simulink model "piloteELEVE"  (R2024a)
settings: Solver=ode45  StartTime=0.0  StopTime=10  RelTol=1e-3  EnableMultiTasking=on
PreLoadFcn:
  | M=0
InitFcn:
  | modelename = gcs
  | path = strcat(modelename,'/mecanisme pilote/Mass')
  | if M==0
  |     set_param(path,'Commented','on')
  | else
  |     set_param(path,'Commented','off')
  | end
libraries: fl_lib x15, nesl_utility x4, sdl_lib x1

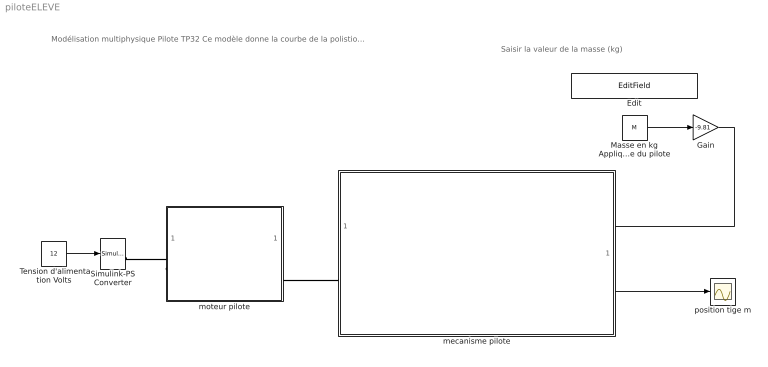
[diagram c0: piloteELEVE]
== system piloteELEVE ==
  note: Saisir la valeur de la masse (kg)
  note: Modélisation multiphysique Pilote TP32 Ce modèle donne la courbe de la polistion de la tige du pilote pendant son mouvement de sortie. Vous pouvez modifier la charge sur la motorisation du pilote en modifiant la valeur de la masse appliquée sur la tige du pilote. Vous devez modifier les paramètres pour que le modèle soit conforme au système.
  " Tension d'alimentation Volts" : Constant  Value=12
  Edit : EditField  LabelPosition=Hide  ShowInitialText=on  Alignment=Center
  Gain : Gain  Gain=-9.81
  Masse en kg Appliquée sur la tige en sortie du pilote : Constant  Value=M
  Simulink-PS Converter : nesl_utility/Simulink-PS Converter  PhysicalDomain=network_engine_domain  SubClassName=ps_input  LeftPortType=input  RightPortType=output  PseudoPeriodic=off  Frequencies=[]  NoiseDistribution=none  NoiseParameters=[]  Unit=1  AffineConversion=off  FilteringAndDerivatives=zero  SimscapeFilterOrder=1  InputFilterTimeConstant=0.001  UdotUserProvided=1
  mecanisme pilote : Subsystem
  moteur pilote : Subsystem
  position tige m : Scope
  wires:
  " Tension d'alimentation Volts"/1 -> Simulink-PS Converter/1
  mecanisme pilote/1(position tige) -> position tige m/1
  Masse en kg Appliquée sur la tige en sortie du pilote/1 -> Gain/1
  Gain/1 -> mecanisme pilote/1(Masse accrochée sur la tige)
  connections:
  moteur pilote/LConn1 -- Simulink-PS Converter/RConn1
  moteur pilote/RConn1 -- mecanisme pilote/LConn1

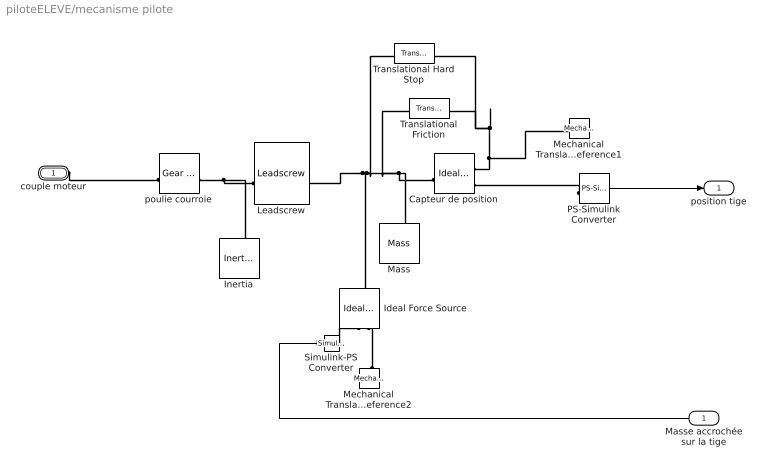
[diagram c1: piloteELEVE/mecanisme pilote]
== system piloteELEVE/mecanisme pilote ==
  Masse accrochée sur la tige : Inport
  Capteur de position : fl_lib/Mechanical/Mechanical Sensors/Ideal Translational Motion Sensor  reference=foundation.enum.MeasurementReference.difference  acceleration_port=false  velocity_port=true  position_port=true  offset=0 mm
  Ideal Force Source : fl_lib/Mechanical/Mechanical Sources/Ideal Force Source
  Inertia : fl_lib/Mechanical/Rotational Elements/Inertia  inertia=0.0005 kg*m^2  num_ports=foundation.enum.numPorts2.one  w_specify=off  w_priority=High  w=0 rad/s  w_nominal_specify=off  w_nominal_value=1  w_nominal_unit=rad/s  t_specify=off  t_priority=None  t=0 N*m  t_nominal_specify=off  t_nominal_value=1  t_nominal_unit=N*m
  Leadscrew : sdl_lib/Gears/Rotational- Translational/Leadscrew  Lead=0.001 m  helix_type=sdl.enum.handedness.right  friction_model=sdl.enum.gear_friction.constant  friction_parameterization=sdl.enum.frictionParameterization.geometry  lambda=15 deg  alpha=14.5 deg  fr_coeff=0.25  eff_sn=0.75  eff_ns=0.45  temperature_TLU=[280, 300, 320] K  efficiency_sn_TLU=[.75, .65, .6]  efficiency_ns_TLU=[.5, .45, .4]  pwr_thr=0.001 W  mu_visc=0.0008 N*m*s/rad  thermal_mass=50 J/K  temperature_specify=off  temperature_priority=High  temperature=300 K  temperature_nominal_specify=off  temperature_nominal_value=1  temperature_nominal_unit=K
  Mass : fl_lib/Mechanical/Translational Elements/Mass  mass=M kg  num_ports=foundation.enum.numPorts2.one  v_specify=off  v_priority=High  v=0 m/s  v_nominal_specify=off  v_nominal_value=1  v_nominal_unit=m/s  f_specify=off  f_priority=None  f=0 N  f_nominal_specify=off  f_nominal_value=1  f_nominal_unit=N
  Mechanical Translational Reference1 : fl_lib/Mechanical/Translational Elements/Mechanical Translational Reference
  Mechanical Translational Reference2 : fl_lib/Mechanical/Translational Elements/Mechanical Translational Reference
  PS-Simulink Converter : nesl_utility/PS-Simulink Converter  PhysicalDomain=network_engine_domain  SubClassName=ps_output  LeftPortType=input  RightPortType=output  PseudoPeriodic=off  Frequencies=[]  VectorFormat=1-D array  Unit=m  AffineConversion=off
  Simulink-PS Converter : nesl_utility/Simulink-PS Converter  PhysicalDomain=network_engine_domain  SubClassName=ps_input  LeftPortType=input  RightPortType=output  PseudoPeriodic=off  Frequencies=[]  NoiseDistribution=none  NoiseParameters=[]  Unit=1  AffineConversion=off  FilteringAndDerivatives=provide  SimscapeFilterOrder=1  InputFilterTimeConstant=0.001  UdotUserProvided=0
  Translational Friction : fl_lib/Mechanical/Translational Elements/Translational Friction  brkwy_frc=15 N  brkwy_vel=0.1 m/s  Col_frc=5 N  visc_coef=30 N*s/m  v_specify=off  v_priority=None  v=0 m/s  v_nominal_specify=off  v_nominal_value=1  v_nominal_unit=m/s  f_specify=off  f_priority=None  f=0 N  f_nominal_specify=off  f_nominal_value=1  f_nominal_unit=N
  Translational Hard Stop : fl_lib/Mechanical/Translational Elements/Translational Hard Stop  upper_bnd=0.250 m  lower_bnd=0 m  model=3  stiff_up=1e6 N/m  stiff_low=1e6 N/m  D_up=150 N/(m/s)  D_low=150 N/(m/s)  transition=0.1 mm  coeff_rest=0.7  v_tol=0.001 m/s  f_tol=0.001 N  v_specify=off  v_priority=None  v=0 m/s  v_nominal_specify=off  v_nominal_value=1  v_nominal_unit=m/s  f_specify=off  f_priority=None  f=0 N  f_nominal_specify=off  f_nominal_value=1  f_nominal_unit=N  x_specify=on  x_priority=High  x=0 m  x_nominal_specify=off  x_nominal_value=1  x_nominal_unit=m  M_specify=off  M_priority=None  M=0
  poulie courroie : fl_lib/Mechanical/Mechanisms/Gear Box  ratio=1  t_in_specify=off  t_in_priority=None  t_in=0 N*m  t_in_nominal_specify=off  t_in_nominal_value=1  t_in_nominal_unit=N*m  t_out_specify=off  t_out_priority=None  t_out=0 N*m  t_out_nominal_specify=off  t_out_nominal_value=1  t_out_nominal_unit=N*m
  couple moteur : PMIOPort  Side=Left
  position tige : Outport
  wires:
  PS-Simulink Converter/1 -> position tige/1
  Masse accrochée sur la tige/1 -> Simulink-PS Converter/1
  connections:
  Capteur de position/RConn1 -- Translational Friction/RConn1 -- Translational Hard Stop/RConn1 -- Mechanical Translational Reference1/LConn1
  Ideal Force Source/LConn1 -- Leadscrew/RConn1 -- Translational Hard Stop/LConn1 -- Translational Friction/LConn1 -- Capteur de position/LConn1 -- Mass/LConn1
  couple moteur/RConn1 -- poulie courroie/LConn1
  PS-Simulink Converter/LConn1 -- Capteur de position/RConn3
  poulie courroie/RConn1 -- Inertia/LConn1 -- Leadscrew/LConn1
  Simulink-PS Converter/RConn1 -- Ideal Force Source/RConn1
  Mechanical Translational Reference2/LConn1 -- Ideal Force Source/RConn2

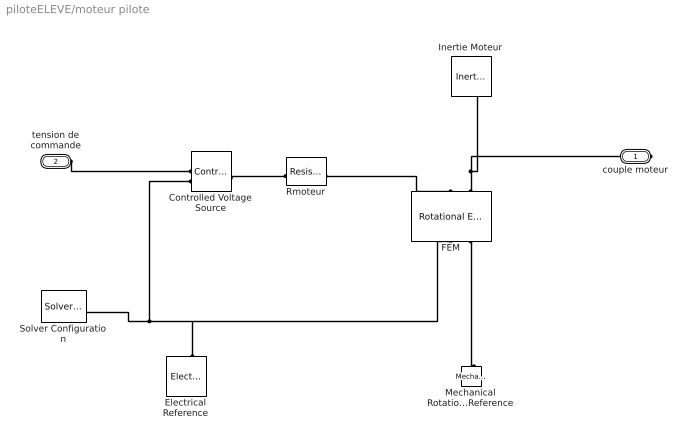
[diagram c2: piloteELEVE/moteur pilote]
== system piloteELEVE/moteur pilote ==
  Controlled Voltage Source : fl_lib/Electrical/Electrical Sources/Controlled Voltage Source
  Electrical Reference : fl_lib/Electrical/Electrical Elements/Electrical Reference
  FEM : fl_lib/Electrical/Electrical Elements/Rotational Electromechanical Converter  K=0.0221 V/(rad/s)  i_specify=off  i_priority=None  i=0 A  i_nominal_specify=off  i_nominal_value=1  i_nominal_unit=A  v_specify=off  v_priority=None  v=0 V  v_nominal_specify=off  v_nominal_value=1  v_nominal_unit=V  t_specify=off  t_priority=None  t=0 N*m  t_nominal_specify=off  t_nominal_value=1  t_nominal_unit=N*m  w_specify=off  w_priority=None  w=0 rad/s  w_nominal_specify=off  w_nominal_value=1  w_nominal_unit=rad/s
  Inertie Moteur : fl_lib/Mechanical/Rotational Elements/Inertia  inertia=0.0000026 kg*m^2  num_ports=foundation.enum.numPorts2.one  w_specify=on  w_priority=High  w=0 rad/s  w_nominal_specify=off  w_nominal_value=1  w_nominal_unit=rad/s  t_specify=off  t_priority=None  t=0 N*m  t_nominal_specify=off  t_nominal_value=1  t_nominal_unit=N*m
  Mechanical Rotational Reference : fl_lib/Mechanical/Rotational Elements/Mechanical Rotational Reference
  Rmoteur : fl_lib/Electrical/Electrical Elements/Resistor  R=0.8 Ohm  i_specify=off  i_priority=None  i=0 A  i_nominal_specify=off  i_nominal_value=1  i_nominal_unit=A  v_specify=off  v_priority=None  v=0 V  v_nominal_specify=off  v_nominal_value=1  v_nominal_unit=V
  Solver Configuration : nesl_utility/Solver Configuration  PhysicalDomain=network_engine_domain  SubClassName=solver  LeftPortType=input  RightPortType=generic  Tones=[]  Harmonics=[]  SimulateNoise=off  Profile=off  UseLocalSampling=off  EnableSwitchedLinearOptims=on  FrequencyDomain=off  UseCCode=off  RelTol=0.001  AbsTol=1e-06  MinStep=1e-09  ToWorkspace=off  RevertToSquareIcSolve=off  NumHomotopyIterations=100  PhasorMode=off  PhasorModeNumHarmonics=1  ConsistencySolver=NEWTON_FTOL  IndexReductionMethod=DerivativeReplacement  DoDC=off  ResidualTolerance=1e-09  ConsistencyTolSource=GLOBAL  ConsistencyAbsTol=0.001  ConsistencyRelTol=0.001  ConsistencyTolFactor=0.001  UseLocalSolver=off  LocalSolverChoice=NE_BACKWARD_EULER_ADVANCER  ResolveIndetEquations=on  FunctionEvalNumThread=1  LocalSolverSampleTime=0.001  DoFixedCost=off  MaxNonlinIter=3  MaxModeIter=2  ComputeImpulses=off  ImpulseIterations=2  LinearAlgebra=Sparse  LinearAlgebraNumThread=0  EquationFormulation=NE_TIME_EF  DelaysMemoryBudget=1024  AutomaticFiltering=on  FilteringTimeConstant=0.001  PartitionStorageMethod=AS_NEEDED  PartitionMemoryBudget=1024  PartitionMethod=FAST  MultibodyUseLocalSolver=off  MultibodyLocalSolverChoice=ODE1  MultibodyLocalSolverSampleTime=0.001
  couple moteur : PMIOPort  Side=Right
  tension de commande : PMIOPort  Port=2  Side=Left
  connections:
  Controlled Voltage Source/LConn1 -- Rmoteur/LConn1
  FEM/LConn2 -- Inertie Moteur/LConn1 -- couple moteur/RConn1
  tension de commande/RConn1 -- Controlled Voltage Source/RConn1
  Electrical Reference/LConn1 -- Solver Configuration/RConn1 -- Controlled Voltage Source/RConn2 -- FEM/RConn1
  FEM/RConn2 -- Mechanical Rotational Reference/LConn1
  Rmoteur/RConn1 -- FEM/LConn1
